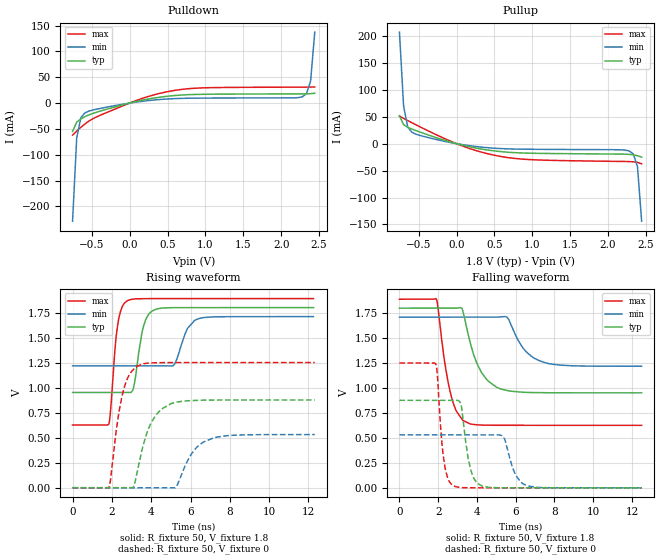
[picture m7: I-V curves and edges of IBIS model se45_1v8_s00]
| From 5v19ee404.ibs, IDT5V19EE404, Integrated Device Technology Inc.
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[Model]   se45_1v8_s00
Model_type   Output
Polarity   Non-Inverting
|   typ   min   max
C_comp   2pF   1.5pF   2.5pF
Vmeas = 0.9V
Rref = 50
Cref = 0
Vref = 0.9V
|   typ   min   max
[Voltage range]   1.8V   1.71V   1.89V
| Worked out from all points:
|   slope of the pulldown table from 0 to 0.27 V, typ, clamps not added: 32 ohm
|   slope of the pullup table from 0 to 0.27 V, typ, clamps not added: 31.6 ohm
|   rising waveform, R_fixture 50, V_fixture 1.8: 20-80 % time 425ps typ, 575ps min, 329ps max; typ from 0.952 V to 1.8 V
|   falling waveform, R_fixture 50, V_fixture 1.8: 20-80 % time 926ps typ, 1.02ns min, 641ps max; typ from 1.8 V to 0.952 V
|   rising waveform, R_fixture 50, V_fixture 0: 20-80 % time 847ps typ, 942ps min, 594ps max; typ from 0 V to 0.877 V
|   falling waveform, R_fixture 50, V_fixture 0: 20-80 % time 416ps typ, 552ps min, 316ps max; typ from 0.877 V to 0 V
[Pulldown]
|Voltage   I (typ)   I (min)   I (max)
|Note, modeling breaks down at 250mA and above.  This is well beyond the functional   |
|operating range of the device.  Should this scenario occur, catastrophic failure and   |
|possible damage to the device and/or board is of higher concern than the I-V curve   |
|behavior.  The IBIS checker will flag currents in excess of 10A with warnings.  Lines   |
|with currents in excess of 0.35 A have been commented out.  The points still remain|
|available to the user if the user desires to use them.   |
|-1.80000e+00   -2.52572e+01   -2.08112e+01   -3.26463e+01
|-1.74490e+00   -2.36799e+01   -1.95979e+01   -3.04476e+01
|-1.68980e+00   -2.21059e+01   -1.83872e+01   -2.82531e+01
|-1.63469e+00   -2.05356e+01   -1.71794e+01   -2.60635e+01
|-1.57959e+00   -1.89696e+01   -1.59750e+01   -2.38796e+01
|-1.52449e+00   -1.74087e+01   -1.47744e+01   -2.17024e+01
|-1.46939e+00   -1.58536e+01   -1.35783e+01   -1.95332e+01
|-1.41429e+00   -1.43055e+01   -1.23874e+01   -1.73739e+01
|-1.35918e+00   -1.27659e+01   -1.12027e+01   -1.52269e+01
|-1.30408e+00   -1.12368e+01   -1.00254e+01   -1.30956e+01
|-1.24898e+00   -9.72098e+00   -8.85722e+00   -1.09851e+01
|-1.19388e+00   -8.22246e+00   -7.70043e+00   -8.90351e+00
|-1.13878e+00   -6.74727e+00   -6.55830e+00   -6.86403e+00
|-1.08367e+00   -5.30512e+00   -5.43552e+00   -4.89135e+00
|-1.02857e+00   -3.91270e+00   -4.33946e+00   -3.03736e+00
|-9.73469e-01   -2.60169e+00   -3.28214e+00   -1.43100e+00
|-9.18367e-01   -1.43880e+00   -2.28475e+00   -3.94093e-01
|-8.63265e-01   -5.66865e-01   -1.38741e+00   -1.06939e-01
|-8.08163e-01   -1.52138e-01   -6.66903e-01   -7.19895e-02
-753.1mV  -54.82mA   -228.9mA   -62.01mA
-698mV    -36.89mA   -66.92mA   -54.09mA
-642.9mV  -30.52mA   -28.08mA   -46.79mA
-587.8mV  -26.13mA   -18.74mA   -40.17mA
-422.4mV  -17.04mA   -11.39mA   -25.78mA
73.47mV   2.606mA    1.636mA    4.206mA
569.4mV   14.28mA    8.482mA    23.96mA
1.01V     17.09mA    9.709mA    29.63mA
2.278V    17.85mA    12.06mA    30.89mA
2.333V    17.94mA    17.98mA    30.92mA
2.388V    18.19mA    42.4mA     30.98mA
2.443V    19.06mA    137.5mA    31.13mA
| 2.49796e+00   2.27208e-02   3.74787e-01   3.15041e-02
| 2.55306e+00   4.08756e-02   7.43068e-01   3.22551e-02
| 2.60816e+00   1.37566e-01   1.19023e+00   3.34916e-02
| 2.66327e+00   4.37819e-01   1.68221e+00   3.56718e-02
| 2.71837e+00   9.27501e-01   2.20139e+00   4.47213e-02
| 2.77347e+00   1.51885e+00   2.73835e+00   1.23384e-01
| 2.82857e+00   2.16314e+00   3.28769e+00   4.92594e-01
| 2.88367e+00   2.83803e+00   3.84607e+00   1.15125e+00
| 2.93878e+00   3.53242e+00   4.41129e+00   1.94102e+00
| 2.99388e+00   4.24015e+00   4.98190e+00   2.79125e+00
| 3.04898e+00   4.95754e+00   5.55682e+00   3.67438e+00
| 3.10408e+00   5.68219e+00   6.13525e+00   4.57781e+00
| 3.15918e+00   6.41253e+00   6.71663e+00   5.49491e+00
| 3.21429e+00   7.14740e+00   7.30048e+00   6.42176e+00
| 3.26939e+00   7.88598e+00   7.88646e+00   7.35591e+00
| 3.32449e+00   8.62763e+00   8.47428e+00   8.29574e+00
| 3.37959e+00   9.37188e+00   9.06370e+00   9.24008e+00
| 3.43469e+00   1.01184e+01   9.65453e+00   1.01881e+01
| 3.48980e+00   1.08667e+01   1.02466e+01   1.11392e+01
| 3.54490e+00   1.16168e+01   1.08398e+01   1.20928e+01
| 3.60000e+00   1.23684e+01   1.14340e+01   1.30487e+01
[Pullup]
|Voltage   I (typ)   I (min)   I (max)
|Note, modeling breaks down at 250mA and above.  This is well beyond the functional   |
|operating range of the device.  Should this scenario occur, catastrophic failure and   |
|possible damage to the device and/or board is of higher concern than the I-V curve   |
|behavior.  The IBIS checker will flag currents in excess of 10A with warnings.  Lines   |
|with currents in excess of 0.35 A have been commented out.  The points still remain|
|available to the user if the user desires to use them.   |
|-1.80000e+00   1.23492e+01   1.04530e+01   1.45809e+01
|-1.74490e+00   1.15979e+01   9.86061e+00   1.36224e+01
|-1.68980e+00   1.08480e+01   9.26940e+00   1.26656e+01
|-1.63469e+00   1.00998e+01   8.67956e+00   1.17108e+01
|-1.57959e+00   9.35349e+00   8.09124e+00   1.07584e+01
|-1.52449e+00   8.60944e+00   7.50468e+00   9.80872e+00
|-1.46939e+00   7.86800e+00   6.92013e+00   8.86233e+00
|-1.41429e+00   7.12967e+00   6.33794e+00   7.91994e+00
|-1.35918e+00   6.39506e+00   5.75851e+00   6.98248e+00
|-1.30408e+00   5.66501e+00   5.18238e+00   6.05131e+00
|-1.24898e+00   4.94068e+00   4.61027e+00   5.12833e+00
|-1.19388e+00   4.22372e+00   4.04313e+00   4.21650e+00
|-1.13878e+00   3.51650e+00   3.48228e+00   3.32063e+00
|-1.08367e+00   2.82280e+00   2.92962e+00   2.44927e+00
|-1.02857e+00   2.14888e+00   2.38803e+00   1.61954e+00
|-9.73469e-01   1.50615e+00   1.86206e+00   8.71510e-01
|-9.18367e-01   9.17564e-01   1.35944e+00   3.11233e-01
|-8.63265e-01   4.33414e-01   8.94316e-01   8.94593e-02
|-8.08163e-01   1.42396e-01   4.94089e-01   5.74619e-02
-753.1mV  52mA       207.1mA    51.2mA
-698mV    35.06mA    69.7mA     46.91mA
-642.9mV  30.25mA    30.46mA    42.81mA
-587.8mV  27.07mA    20.93mA    38.78mA
-312.2mV  13.24mA    9.215mA    19.54mA
73.47mV   -2.62mA    -1.732mA   -4.049mA
569.4mV   -14.56mA   -9.029mA   -23.39mA
1.065V    -17.95mA   -10.52mA   -30.19mA
2.278V    -19.91mA   -13.47mA   -33.25mA
2.333V    -20.75mA   -19.16mA   -33.68mA
2.388V    -22.37mA   -42.35mA   -34.85mA
2.443V    -25.08mA   -144mA     -37.25mA
| 2.49796e+00   -3.03122e-02   -4.72515e-01   -4.09753e-02
| 2.55306e+00   -4.85503e-02   -1.10341e+00   -4.57713e-02
| 2.60816e+00   -1.49867e-01   -1.94886e+00   -5.14012e-02
| 2.66327e+00   -5.72739e-01   -2.91646e+00   -5.79887e-02
| 2.71837e+00   -1.45030e+00   -3.95533e+00   -7.00790e-02
| 2.77347e+00   -2.61576e+00   -5.03908e+00   -1.50146e-01
| 2.82857e+00   -3.92793e+00   -6.15313e+00   -6.90731e-01
| 2.88367e+00   -5.32086e+00   -7.28879e+00   -1.99805e+00
| 2.93878e+00   -6.76320e+00   -8.44055e+00   -3.72340e+00
| 2.99388e+00   -8.23838e+00   -9.60470e+00   -5.63149e+00
| 3.04898e+00   -9.73678e+00   -1.07787e+01   -7.63318e+00
| 3.10408e+00   -1.12524e+01   -1.19607e+01   -9.69020e+00
| 3.15918e+00   -1.27812e+01   -1.31493e+01   -1.17833e+01
| 3.21429e+00   -1.43206e+01   -1.43434e+01   -1.39018e+01
| 3.26939e+00   -1.58683e+01   -1.55422e+01   -1.60388e+01
| 3.32449e+00   -1.74231e+01   -1.67451e+01   -1.81901e+01
| 3.37959e+00   -1.89838e+01   -1.79514e+01   -2.03526e+01
| 3.43469e+00   -2.05494e+01   -1.91609e+01   -2.25242e+01
| 3.48980e+00   -2.21193e+01   -2.03730e+01   -2.47033e+01
| 3.54490e+00   -2.36930e+01   -2.15876e+01   -2.68887e+01
| 3.60000e+00   -2.52699e+01   -2.28044e+01   -2.90795e+01
[Ramp]
|   typ   min   max
dV/dt_r   0.509/0.425n   0.296/0.576n   0.758/0.329n
dV/dt_f   0.512/0.927n   0.298/1.018n   0.761/0.641n
R_load =   50.0000
[Rising Waveform]
R_fixture = 50
V_fixture = 1.8   |Vcc_typ
V_fixture_min = 1.71 |Vcc_min
V_fixture_max = 1.89 |Vcc_max
C_fixture = 0.0p
| Time   typ   min   max
0s        951.9mV    1.218V     626.3mV
1.838ns   951.9mV    1.218V     632.2mV
2.302ns   951.9mV    1.218V     1.633V
2.799ns   951.3mV    1.218V     1.87V
3.081ns   981.7mV    1.218V     1.884V
3.714ns   1.677V     1.218V     1.89V
4.262ns   1.785V     1.218V     1.89V
5.14ns    1.8V       1.224V     1.89V
6.422ns   1.8V       1.69V      1.89V
12.26ns   1.8V       1.71V      1.89V
[Falling Waveform]
R_fixture = 50
V_fixture = 1.8   |Vcc_typ
V_fixture_min = 1.71 |Vcc_min
V_fixture_max = 1.89 |Vcc_max
C_fixture = 0.0p
| Time   typ   min   max
0s        1.8V       1.71V      1.89V
1.889ns   1.8V       1.71V      1.896V
2.57ns    1.8V       1.71V      1.004V
3.269ns   1.776V     1.71V      676.1mV
4.048ns   1.226V     1.71V      630.8mV
5ns       1.009V     1.71V      626.9mV
5.543ns   975.6mV    1.711V     626.6mV
6.465ns   956.9mV    1.38V      626.5mV
7.5ns     952.8mV    1.254V     626.5mV
12.5ns    951.9mV    1.218V     626.4mV
[Rising Waveform]
R_fixture = 50
V_fixture = 0
C_fixture = 0.0p
| Time   typ   min   max
0s        62.71nV    55.96nV    63.02nV
1.847ns   96.85nV    55.94nV    -997.8uV
2.5ns     -246.3nV   55.94nV    901.4mV
3.079ns   908.7uV    83.32nV    1.178V
3.235ns   108mV      54.26nV    1.21V
3.963ns   634.7mV    -630.9nV   1.247V
5ns       840.1mV    -584uV     1.251V
6.25ns    873.2mV    389.7mV    1.251V
7.12ns    876.2mV    493.3mV    1.251V
12.32ns   876.9mV    531.2mV    1.251V
[Falling Waveform]
R_fixture = 50
V_fixture = 0
C_fixture = 0.0p
| Time   typ   min   max
0s        876.9mV    531.2mV    1.251V
1.891ns   876.9mV    531.2mV    1.234V
2.33ns    876.9mV    531.2mV    232.1mV
2.798ns   877mV      531.2mV    19.61mV
3.179ns   831.6mV    531.2mV    2.311mV
3.75ns    135.8mV    531.2mV    301uV
4.274ns   17.11mV    531.2mV    220.5uV
5.353ns   557.7uV    513.3mV    136.1uV
6.635ns   256.8uV    19.26mV    92.83uV
12.5ns    73.73uV    169.1uV    36.13uV
